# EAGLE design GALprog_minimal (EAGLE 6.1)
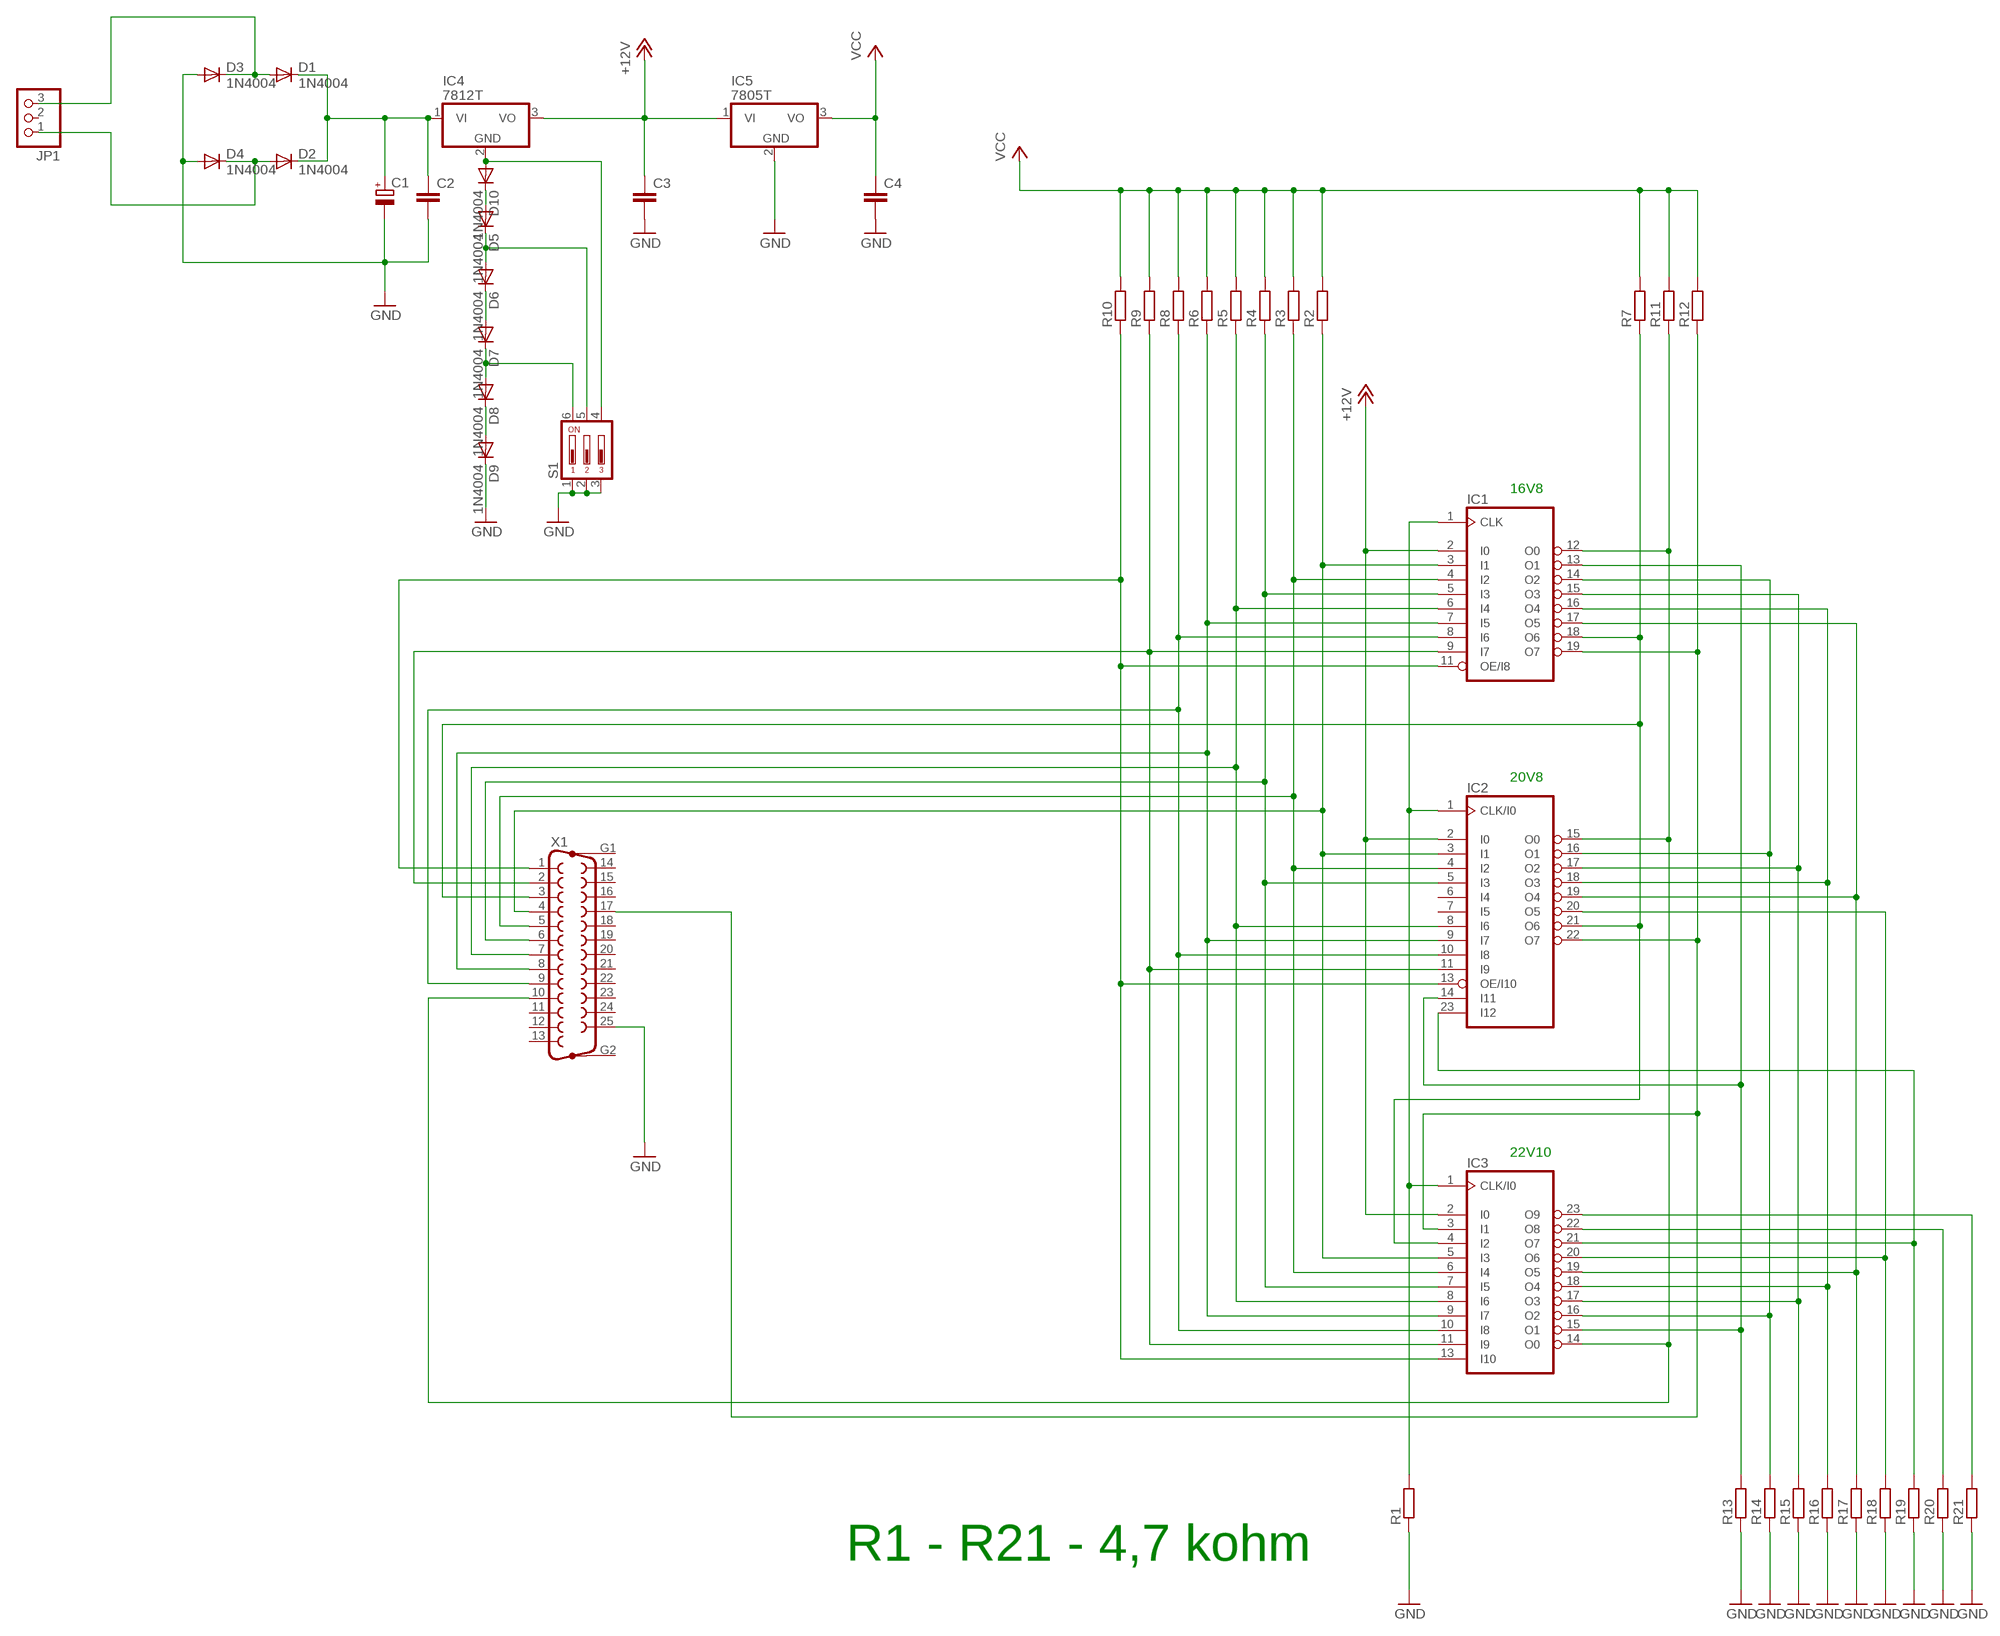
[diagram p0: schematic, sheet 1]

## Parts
C1  CPOL-EUE5-10.5  [E5-10,5]
C2  C-EU050-024X044  [C050-024X044]
C3  C-EU050-024X044  [C050-024X044]
C4  C-EU050-024X044  [C050-024X044]
D1  1N4004  [DO41-10]
D2  1N4004  [DO41-10]
D3  1N4004  [DO41-10]
D4  1N4004  [DO41-10]
D5  1N4004  [DO41-10]
D6  1N4004  [DO41-10]
D7  1N4004  [DO41-10]
D8  1N4004  [DO41-10]
D9  1N4004  [DO41-10]
D10  1N4004  [DO41-10]
IC1  16V8  [DIL20]
IC2  20V8  [DIL24-3]
IC3  22V10  [DIL24-3]
IC4  7812T  [TO220H]
IC5  7805T  [TO220H]
JP1  PINHD-1X3  [1X03]
R1  R-EU_0204/7  [0204/7]
R2  R-EU_0204/7  [0204/7]
R3  R-EU_0204/7  [0204/7]
R4  R-EU_0204/7  [0204/7]
R5  R-EU_0204/7  [0204/7]
R6  R-EU_0204/7  [0204/7]
R7  R-EU_0204/7  [0204/7]
R8  R-EU_0204/7  [0204/7]
R9  R-EU_0204/7  [0204/7]
R10  R-EU_0204/7  [0204/7]
R11  R-EU_0204/7  [0204/7]
R12  R-EU_0204/7  [0204/7]
R13  R-EU_0204/7  [0204/7]
R14  R-EU_0204/7  [0204/7]
R15  R-EU_0204/7  [0204/7]
R16  R-EU_0204/7  [0204/7]
R17  R-EU_0204/7  [0204/7]
R18  R-EU_0204/7  [0204/7]
R19  R-EU_0204/7  [0204/7]
R20  R-EU_0204/7  [0204/7]
R21  R-EU_0204/7  [0204/7]
S1  DP03  [DP-03]
X1  F25HP  [F25HP]

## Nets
+12V: C3.1 IC1.2(I0) IC2.2(I0) IC3.2(I0) IC4.3(VO) IC5.1(VI)
GND: C1.- C2.2 C3.2 C4.2 D3.A D4.A D9.C IC5.2(GND) R1.1 R13.1 R14.1 R15.1 R16.1 R17.1 R18.1 R19.1 R20.1 R21.1 S1.1 S1.2 S1.3 X1.25
N$1: IC1.1(CLK) IC2.1(CLK/I0) IC3.1(CLK/I0) R1.2
N$2: IC1.18(O6) IC2.21(O6) IC3.4(I2) R7.1 X1.3
N$3: IC1.3(I1) IC2.3(I1) IC3.5(I3) R2.1 X1.4
N$4: D2.A D4.C JP1.1
N$5: IC1.6(I4) IC2.8(I6) IC3.8(I6) R5.1 X1.7
N$6: IC1.4(I2) IC2.4(I2) IC3.6(I4) R3.1 X1.5
N$7: D1.A D3.C JP1.3
N$8: D10.A IC4.2(GND) S1.4
N$9: IC1.5(I3) IC2.5(I3) IC3.7(I5) R4.1 X1.6
N$10: C1.+ C2.1 D1.C D2.C IC4.1(VI)
N$11: D5.C D6.A S1.5
N$12: IC1.7(I5) IC2.9(I7) IC3.9(I7) R6.1 X1.8
N$13: D6.C D7.A
N$14: IC1.12(O0) IC2.15(O0) IC3.14(O0) R11.1 X1.10
N$16: D7.C D8.A S1.6
N$17: D8.C D9.A
N$18: D5.A D10.C
N$19: IC1.8(I6) IC2.10(I8) IC3.10(I8) R8.1 X1.9
N$20: IC1.11(OE/I8) IC2.13(OE/I10) IC3.13(I10) R10.1 X1.1
N$21: IC1.19(O7) IC2.22(O7) IC3.3(I1) R12.1 X1.17
N$23: IC1.9(I7) IC2.11(I9) IC3.11(I9) R9.1 X1.2
N$27: IC1.13(O1) IC2.14(I11) IC3.15(O1) R13.2
N$29: IC1.14(O2) IC2.16(O1) IC3.16(O2) R14.2
N$30: IC1.15(O3) IC2.17(O2) IC3.17(O3) R15.2
N$31: IC1.16(O4) IC2.18(O3) IC3.18(O4) R16.2
N$32: IC1.17(O5) IC2.19(O4) IC3.19(O5) R17.2
N$33: IC2.20(O5) IC3.20(O6) R18.2
N$34: IC2.23(I12) IC3.21(O7) R19.2
N$35: IC3.22(O8) R20.2
N$36: IC3.23(O9) R21.2
VCC: C4.1 IC5.3(VO) R2.2 R3.2 R4.2 R5.2 R6.2 R7.2 R8.2 R9.2 R10.2 R11.2 R12.2
Unconnected: IC2.6(I4) IC2.7(I5) JP1.2 X1.11 X1.12 X1.13 X1.14 X1.15 X1.16 X1.18 X1.19 X1.20 X1.21 X1.22 X1.23 X1.24 X1.G1 X1.G2

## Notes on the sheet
- 16V8
- 20V8
- 22V10
- R1 - R21 - 4,7 kohm

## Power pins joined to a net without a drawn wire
GND: IC1.10(GND) IC2.12(GND) IC3.12(GND)
VCC: IC1.20(VCC) IC2.24(VCC) IC3.24(VCC)

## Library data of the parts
C1 = rcl:CPOL-EU: POLARIZED CAPACITOR, European symbol
C2-C4 = rcl:C-EU: CAPACITOR, European symbol
D1-D10 = diode:1N4004: DIODE
IC1 = pal:16V8: PAL; MPN: GAL16V8D-7LPN; OC_FARNELL: 9699740; OC_NEWARK: 97K0449
IC2 = pal:20V8: PAL; MF: FARNELL; MPN: GAL20V8B-25QP; OC_FARNELL: 3327462; OC_NEWARK: 70C8546
IC3 = pal:22V10: PAL; MPN: GAL22V10D-7LPN; OC_FARNELL: 1571925; OC_NEWARK: 97M0480
IC4 IC5 = linear:78*: Positive VOLTAGE REGULATOR Source: http://cache.national.com/ds/LM/LM78L05.pdf http://www.fairchildsemi.com/ds/LM/LM7805.pdf
JP1 = pinhead:PINHD-1X3: PIN HEADER
R1-R21 = rcl:R-EU_: RESISTOR, European symbol
S1 = switch-dil:DP03: DIL/CODE SWITCH; MPN: MCDP03; OC_FARNELL: 1522004; OC_NEWARK: 74M2976
X1 = con-subd:F25HP: SUB-D; OC_FARNELL: unknown; OC_NEWARK: unknown

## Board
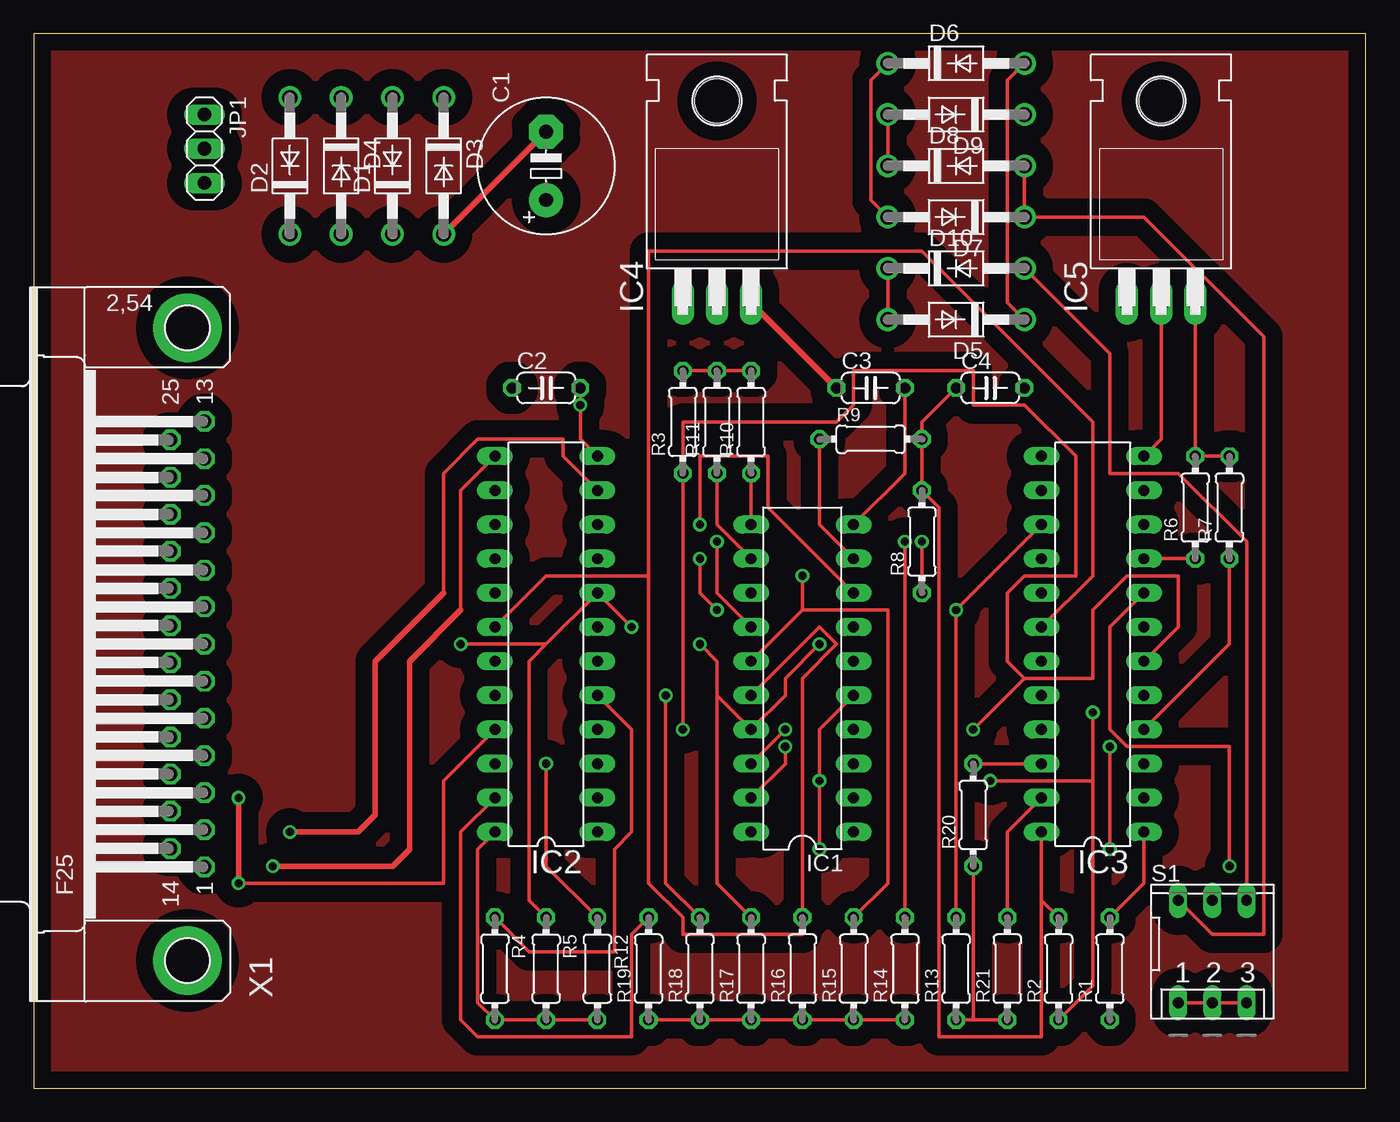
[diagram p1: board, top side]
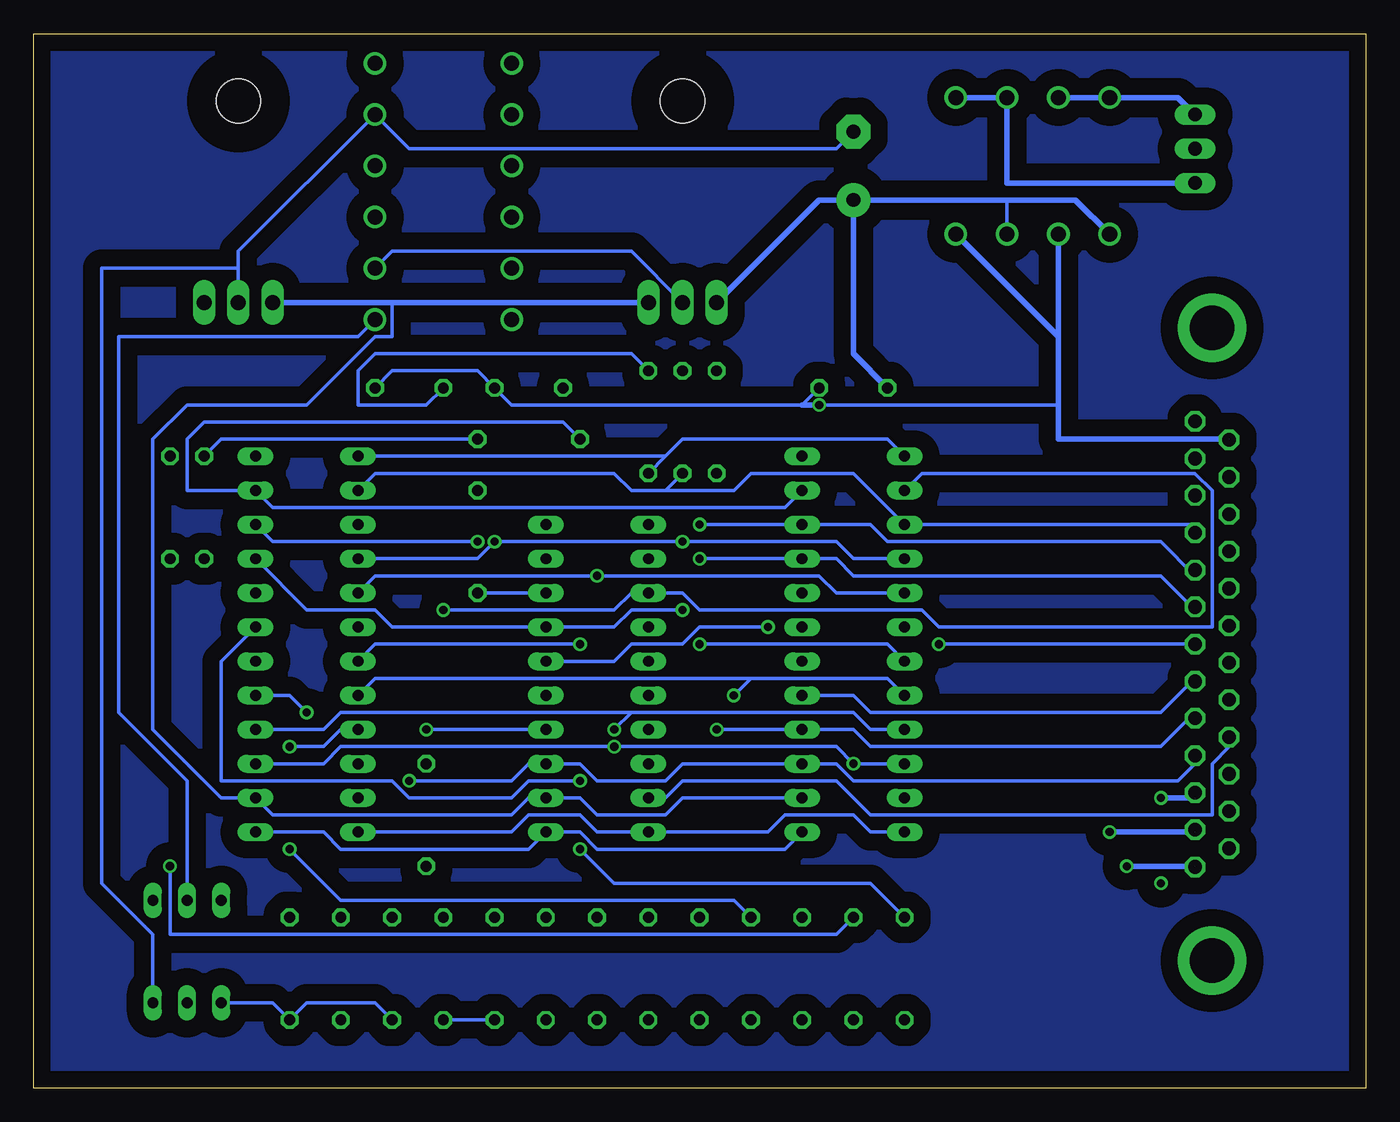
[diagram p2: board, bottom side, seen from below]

Size 99.04 x 78.41 mm. Coordinates in mm from the lower left corner, seen from the top.
Outline: 0,0 99.04,0 99.04,78.41 0,78.41 0,0
Copper layers (1*16): Top 0.035mm / dielectric 1.5mm / Bottom 0.035mm
Design rules: minimum track width 10mil, minimum drill 24mil, track to track 8mil, track to pad 8mil, pad to pad 8mil, via to via 8mil, smd to smd 8mil, copper to edge 40mil, drill to drill 8mil, minimum pad ring 10mil, minimum via ring 8mil, stop-mask expansion 4mil, vias tented up to drill 0mil, thermal gap 10mil

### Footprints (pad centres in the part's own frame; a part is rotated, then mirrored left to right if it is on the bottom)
E5-10,5 = drill 1.016 pad 2.54: + -2.54,0 | drill 1.016 pad 2.54 octagon: - 2.54,0
C050-024X044 = drill 0.813 octagon: 1 -2.54,0; 2 2.54,0
DO41-10 = drill 1.118: A 5.08,0; C -5.08,0
DIL20 = drill 0.813 long: 1 -11.43,-3.81; 2 -8.89,-3.81; 3 -6.35,-3.81; 4 -3.81,-3.81; 5 -1.27,-3.81; 6 1.27,-3.81; 7 3.81,-3.81; 8 6.35,-3.81; 9 8.89,-3.81; 10 11.43,-3.81; 11 11.43,3.81; 12 8.89,3.81; 13 6.35,3.81; 14 3.81,3.81; 15 1.27,3.81; 16 -1.27,3.81; 17 -3.81,3.81; 18 -6.35,3.81; 19 -8.89,3.81; 20 -11.43,3.81
DIL24-3 = drill 0.813 long: 1 -13.97,-3.81; 2 -11.43,-3.81; 3 -8.89,-3.81; 4 -6.35,-3.81; 5 -3.81,-3.81; 6 -1.27,-3.81; 7 1.27,-3.81; 8 3.81,-3.81; 9 6.35,-3.81; 10 8.89,-3.81; 11 11.43,-3.81; 12 13.97,-3.81; 13 13.97,3.81; 14 11.43,3.81; 15 8.89,3.81; 16 6.35,3.81; 17 3.81,3.81; 18 1.27,3.81; 19 -1.27,3.81; 20 -3.81,3.81; 21 -6.35,3.81; 22 -8.89,3.81; 23 -11.43,3.81; 24 -13.97,3.81
TO220H = drill 1.118 long: 1 -2.54,-10.16; 2 0,-10.16; 3 2.54,-10.16 | hole 3.302: 0,4.826
1X03 = drill 1.016 long: 1 -2.54,0; 2 0,0; 3 2.54,0
0204/7 = drill 0.813 octagon: 1 -3.81,0; 2 3.81,0
DP-03 = drill 0.813 long: 1 -2.54,-3.81; 2 0,-3.81; 3 2.54,-3.81; 4 2.54,3.81; 5 0,3.81; 6 -2.54,3.81
F25HP = drill 1.016 octagon: 1 -16.561,-1.27; 2 -13.792,-1.27; 3 -11.049,-1.27; 4 -8.28,-1.27; 5 -5.512,-1.27; 6 -2.769,-1.27; 7 0,-1.27; 8 2.769,-1.27; 9 5.512,-1.27; 10 8.28,-1.27; 11 11.049,-1.27; 12 13.792,-1.27; 13 16.561,-1.27; 14 -15.189,1.27; 15 -12.421,1.27; 16 -9.652,1.27; 17 -6.909,1.27; 18 -4.14,1.27; 19 -1.372,1.27; 20 1.372,1.27; 21 4.14,1.27; 22 6.909,1.27; 23 9.652,1.27; 24 12.421,1.27; 25 15.189,1.27 | drill 3.302 pad 5.08: G1 -23.52,0; G2 23.52,0

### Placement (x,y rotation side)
C1  38.1,68.58 90 top
C2  38.1,52.07 0 top
C3  62.23,52.07 0 top
C4  71.12,52.07 0 top
D1  26.67,68.58 90 top
D2  19.05,68.58 90 top
D3  30.48,68.58 270 top
D4  22.86,68.58 270 top
D5  68.58,57.15 180 top
D6  68.58,76.2 0 top
D7  68.58,64.77 180 top
D8  68.58,68.58 0 top
D9  68.58,72.39 180 top
D10  68.58,60.96 0 top
IC1  57.15,30.48 90 top
IC2  38.1,33.02 90 top
IC3  78.74,33.02 90 top
IC4  50.8,68.58 0 top
IC5  83.82,68.58 0 top
JP1  12.7,69.85 270 top
R1  80.01,8.89 90 top
R2  76.2,8.89 90 top
R3  48.26,49.53 90 top
R4  34.29,8.89 270 top
R5  38.1,8.89 270 top
R6  86.36,43.18 90 top
R7  88.9,43.18 90 top
R8  66.04,40.64 90 top
R9  62.23,48.26 0 top
R10  53.34,49.53 90 top
R11  50.8,49.53 90 top
R12  41.91,8.89 270 top
R13  68.58,8.89 90 top
R14  64.77,8.89 90 top
R15  60.96,8.89 90 top
R16  57.15,8.89 90 top
R17  53.34,8.89 90 top
R18  49.53,8.89 90 top
R19  45.72,8.89 90 top
R20  69.85,20.32 90 top
R21  72.39,8.89 90 top
S1  87.63,10.16 0 top
X1  11.43,33.02 90 top

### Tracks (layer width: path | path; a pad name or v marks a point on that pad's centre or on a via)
+12V
  Top 0.406: IC4.3 C3.1
  Bottom 0.254: IC2.2 50.8,21.59 52.07,20.32 57.15,20.32 58.42,21.59 IC1.2 62.23,21.59 63.5,20.32 81.28,20.32 IC3.2 85.09,21.59 90.17,26.67 90.17,48.26 87.63,50.8 78.74,50.8 73.66,55.88 72.39,55.88 72.39,58.42
  Bottom 0.406: IC4.3 72.39,58.42 IC5.1
GND  (via drill 0.6)  (1 unrouted)
  Top 0.254: R19.1 R18.1 R17.1 R16.1 R15.1 R14.1 | S1.1 S1.2 S1.3 | R21.1 69.85,5.08 | 69.85,5.08 R13.1 | 69.85,5.08 R20.1 | IC3.12 83.82,48.26 IC5.2 | IC1.10 64.77,45.72 C3.2 | IC2.12 40.64,48.26 v40.64,50.8 C2.2 | 10.16,48.26 X1.25
  Top 0.406: D3.A C1.-
  Bottom 0.254: S1.1 81.28,6.35 R1.1 78.74,6.35 73.66,6.35 R21.1 | R13.1 R14.1 | IC5.2 83.82,60.96 | 83.82,60.96 83.82,62.23 D9.C 71.12,69.85 39.37,69.85 C1.- | C4.2 72.39,53.34 66.04,53.34 C3.2 63.5,50.8 41.91,50.8 C2.2 | 22.86,50.8 v40.64,50.8 | S1.3 90.17,11.43 93.98,15.24 93.98,60.96 83.82,60.96
  Bottom 0.406: D4.A 22.86,55.88 | 22.86,55.88 22.86,50.8 22.86,48.26 10.16,48.26 | 22.86,55.88 D3.A | v40.64,50.8 41.91,50.8
N$1
  Top 0.254: R1.2 82.55,15.24 IC3.1
  Bottom 0.254: IC2.1 43.18,17.78 57.15,17.78 58.42,19.05 IC1.1 62.23,17.78 76.2,17.78 77.47,19.05 IC3.1
N$2  (via drill 0.6, 0.61)  (1 unrouted)
  Top 0.254: IC3.4 88.9,33.02 R7.1 | v55.88,26.67 IC1.18 | v15.24,15.24 30.48,15.24 30.48,22.86 IC2.21 | 12.7,21.59 X1.3
  Top 0.406: v15.24,21.59 v15.24,15.24
  Bottom 0.254: 54.61,27.94 v55.88,26.67 | 54.61,27.94 38.1,27.94 36.83,26.67 IC2.21 | IC3.4 77.47,26.67 76.2,27.94 54.61,27.94
  Bottom 0.406: 12.7,21.59 v15.24,21.59
N$3  (via drill 0.61)
  Top 0.254: R2.1 78.74,7.62 78.74,22.86 | v78.74,27.94 78.74,22.86 | v71.12,22.86 78.74,22.86
  Bottom 0.254: v78.74,27.94 80.01,29.21 IC3.5 | X1.4 12.7,24.13 13.97,22.86 38.1,22.86 39.37,24.13 IC2.3 50.8,24.13 52.07,22.86 57.15,22.86 58.42,24.13 IC1.3 62.23,24.13 63.5,22.86 v71.12,22.86
N$4
  Bottom 0.406: JP1.1 13.97,73.66 D2.A D4.C
N$5  (via drill 0.61)
  Top 0.254: R5.1 36.83,13.97 36.83,31.75 38.1,33.02 | 38.1,33.02 IC2.8 v44.45,34.29 | IC3.8 80.01,34.29 80.01,26.67 81.28,25.4 88.9,25.4 v88.9,16.51 | 38.1,33.02 v31.75,33.02
  Bottom 0.254: IC1.6 55.88,31.75 54.61,33.02 50.8,33.02 49.53,34.29 v44.45,34.29 | v88.9,16.51 88.9,11.43 39.37,11.43 R5.1 | v31.75,33.02 X1.7
N$6  (via drill 0.61)
  Top 0.254: 73.66,30.48 v69.85,26.67 | 73.66,30.48 78.74,30.48 78.74,35.56 81.28,38.1 85.09,38.1 85.09,34.29 IC3.6 | v48.26,26.67 R3.1 48.26,49.53 59.69,49.53 60.96,50.8 60.96,53.34 69.85,53.34 69.85,50.8 73.66,50.8 77.47,46.99 77.47,38.1 73.66,38.1 72.39,36.83 72.39,31.75 73.66,30.48
  Bottom 0.254: v69.85,26.67 IC1.4 | X1.5 12.7,27.94 15.24,25.4 36.83,25.4 38.1,26.67 IC2.4 v48.26,26.67
N$7
  Bottom 0.406: JP1.3 26.67,67.31 D1.A D3.C
N$8
  Top 0.254: S1.4 90.17,40.64 85.09,45.72 80.01,45.72 80.01,54.61 D10.A
  Bottom 0.254: IC4.2 54.61,62.23 72.39,62.23 D10.A
N$9  (via drill 0.61)
  Top 0.254: R4.1 36.83,10.16 43.18,10.16 43.18,17.78 44.45,19.05 44.45,26.67 IC2.5 | IC1.5 58.42,26.67 v58.42,22.86 v58.42,17.78
  Bottom 0.254: v58.42,17.78 55.88,15.24 36.83,15.24 R4.1 | IC3.7 85.09,31.75 85.09,22.86 72.39,22.86 71.12,21.59 63.5,21.59 62.23,22.86 v58.42,22.86 | IC2.5 38.1,29.21 36.83,27.94 15.24,27.94 12.7,30.48 X1.6
N$10
  Bottom 0.254: 26.67,66.04 D1.C
  Bottom 0.406: C2.1 38.1,54.61 C1.+ | IC4.1 40.64,66.04 C1.+ | D2.C 21.59,66.04 26.67,66.04 C1.+
N$11
  Top 0.254: D6.A 72.39,74.93 72.39,58.42 D5.C
  Bottom 0.254: S1.5 87.63,22.86 92.71,27.94 92.71,55.88 74.93,55.88 D5.C
N$12  (via drill 0.61)
  Top 0.254: IC3.9 R6.1 | v50.8,35.56 49.53,36.83 v49.53,39.37
  Bottom 0.254: IC3.9 78.74,35.56 73.66,35.56 72.39,34.29 IC1.7 55.88,34.29 54.61,35.56 v50.8,35.56 | X1.8 12.7,35.56 15.24,38.1 38.1,38.1 39.37,39.37 IC2.9 v49.53,39.37
N$13
  Top 0.254: D7.A 62.23,66.04 62.23,74.93 D6.C
N$14
  Top 0.254: IC1.12 50.8,41.91 R11.1
  Bottom 0.254: X1.10 12.7,41.91 IC2.15 38.1,45.72 45.72,45.72 46.99,44.45 52.07,44.45 | IC3.14 73.66,45.72 55.88,45.72 54.61,44.45 52.07,44.45 | R11.1 52.07,44.45
N$15
  pour Bottom (isolate 1.27): 0,78.74 99.06,78.74 99.06,0 0,0
N$16
  Top 0.254: S1.6 87.63,11.43 91.44,11.43 91.44,55.88 82.55,64.77 D7.C D8.A
N$17
  Top 0.254: D9.A D8.C
N$18
  Top 0.254: D10.C D5.A
N$19  (via drill 0.61)
  Top 0.254: R8.1 v66.04,40.64 | IC1.8 54.61,43.18 54.61,46.99 49.53,46.99 v49.53,41.91
  Bottom 0.254: R8.1 IC1.8 | IC3.10 81.28,40.64 v66.04,40.64 | X1.9 12.7,38.1 15.24,40.64 35.56,40.64 36.83,41.91 IC2.10 v49.53,41.91
N$20  (via drill 0.6)  (1 unrouted)
  Top 0.254: R10.1 IC1.11 | 31.75,35.56 31.75,44.45 IC2.13 | 12.7,16.51 X1.1
  Top 0.406: 31.75,35.56 27.94,31.75 27.94,17.78 26.67,16.51 v17.78,16.51
  Bottom 0.254: IC2.13 35.56,48.26 50.8,48.26 52.07,46.99 | R10.1 52.07,46.99 | 52.07,46.99 IC3.13
  Bottom 0.406: 12.7,16.51 v17.78,16.51
N$21  (via drill 0.61)
  Top 0.254: R12.1 38.1,16.51 v38.1,24.13 | IC1.19 55.88,24.13 v55.88,25.4
  Bottom 0.254: IC2.22 v38.1,24.13 39.37,25.4 v55.88,25.4 76.2,25.4 77.47,24.13 IC3.3 | IC1.19 52.07,21.59 50.8,22.86 39.37,22.86 36.83,20.32 11.43,20.32 11.43,24.13 10.16,25.4 X1.17
N$22
  pour Top (isolate 1.27): 0,78.74 99.06,78.74 99.06,0 0,0
N$23  (via drill 0.6)  (1 unrouted)
  Top 0.254: R9.1 58.42,41.91 IC1.9 | 30.48,36.83 30.48,45.72 33.02,48.26 39.37,48.26 39.37,46.99 IC2.11 | 12.7,19.05 X1.2
  Top 0.406: 30.48,36.83 25.4,31.75 25.4,20.32 24.13,19.05 v19.05,19.05
  Bottom 0.254: IC2.11 43.18,43.18 81.28,43.18 IC3.11 87.63,44.45 87.63,48.26 86.36,49.53 59.69,49.53 R9.1
  Bottom 0.406: 12.7,19.05 v19.05,19.05
N$27  (via drill 0.61)
  Top 0.254: R13.2 v68.58,35.56 IC3.15
  Bottom 0.254: IC2.14 33.02,45.72 12.7,45.72 11.43,44.45 11.43,34.29 31.75,34.29 33.02,35.56 49.53,35.56 50.8,36.83 IC1.13 54.61,36.83 55.88,35.56 v68.58,35.56
N$29  (via drill 0.61)
  Top 0.254: IC1.14 50.8,36.83 v50.8,40.64 | v64.77,40.64 R14.2
  Bottom 0.254: IC2.16 38.1,39.37 39.37,40.64 v50.8,40.64 v64.77,40.64 66.04,39.37 IC3.16
N$30  (via drill 0.61)
  Top 0.254: 57.15,35.56 IC1.15 | 57.15,35.56 63.5,35.56 63.5,15.24 R15.2 | v57.15,38.1 57.15,35.56
  Bottom 0.254: IC2.17 39.37,36.83 40.64,38.1 v57.15,38.1 73.66,38.1 IC3.17
N$31
  Top 0.254: IC2.18 38.1,38.1 45.72,38.1 | 45.72,38.1 45.72,15.24 48.26,12.7 48.26,11.43 57.15,11.43 R16.2 57.15,30.48 59.69,33.02 58.42,34.29 IC1.16 | IC3.18 78.74,38.1 78.74,49.53 66.04,62.23 45.72,62.23 45.72,38.1
N$32  (via drill 0.61)
  Top 0.254: v49.53,33.02 50.8,31.75 50.8,29.21 | 50.8,29.21 IC1.17 55.88,29.21 55.88,30.48 v58.42,33.02 | R17.2 50.8,15.24 50.8,29.21
  Bottom 0.254: IC2.19 35.56,33.02 v49.53,33.02 | IC3.19 73.66,33.02 v58.42,33.02
N$33  (via drill 0.61)
  Top 0.254: R18.2 46.99,15.24 v46.99,29.21
  Bottom 0.254: 45.72,30.48 v46.99,29.21 | 45.72,30.48 35.56,30.48 IC2.20 | IC3.20 73.66,30.48 45.72,30.48
N$34  (via drill 0.61)
  Top 0.254: IC2.23 31.75,19.05 31.75,5.08 33.02,3.81 44.45,3.81 44.45,11.43 R19.2 | v80.01,17.78 v80.01,25.4
  Bottom 0.254: IC3.21 76.2,26.67 77.47,25.4 v80.01,25.4 | v80.01,17.78 76.2,13.97 46.99,13.97 R19.2
N$35
  Top 0.254: IC3.22 R20.2
N$36
  Top 0.254: R21.2 72.39,19.05 IC3.23
VCC
  Top 0.254: R7.2 R6.2 IC5.3 | R3.2 R11.2 R10.2 | C4.1 66.04,49.53 R9.2 R8.2 67.31,43.18 67.31,3.81 74.93,3.81 74.93,13.97 | 74.93,13.97 R2.2 | IC3.24 74.93,13.97 | R12.2 R5.2 R4.2 33.02,6.35 33.02,17.78 IC2.24
  Bottom 0.254: R10.2 54.61,54.61 73.66,54.61 74.93,53.34 74.93,50.8 69.85,50.8 C4.1 | R6.2 85.09,48.26 R9.2 | IC2.24 36.83,19.05 38.1,20.32 43.18,20.32 44.45,19.05 IC1.20 57.15,19.05 58.42,20.32 62.23,20.32 63.5,19.05 IC3.24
